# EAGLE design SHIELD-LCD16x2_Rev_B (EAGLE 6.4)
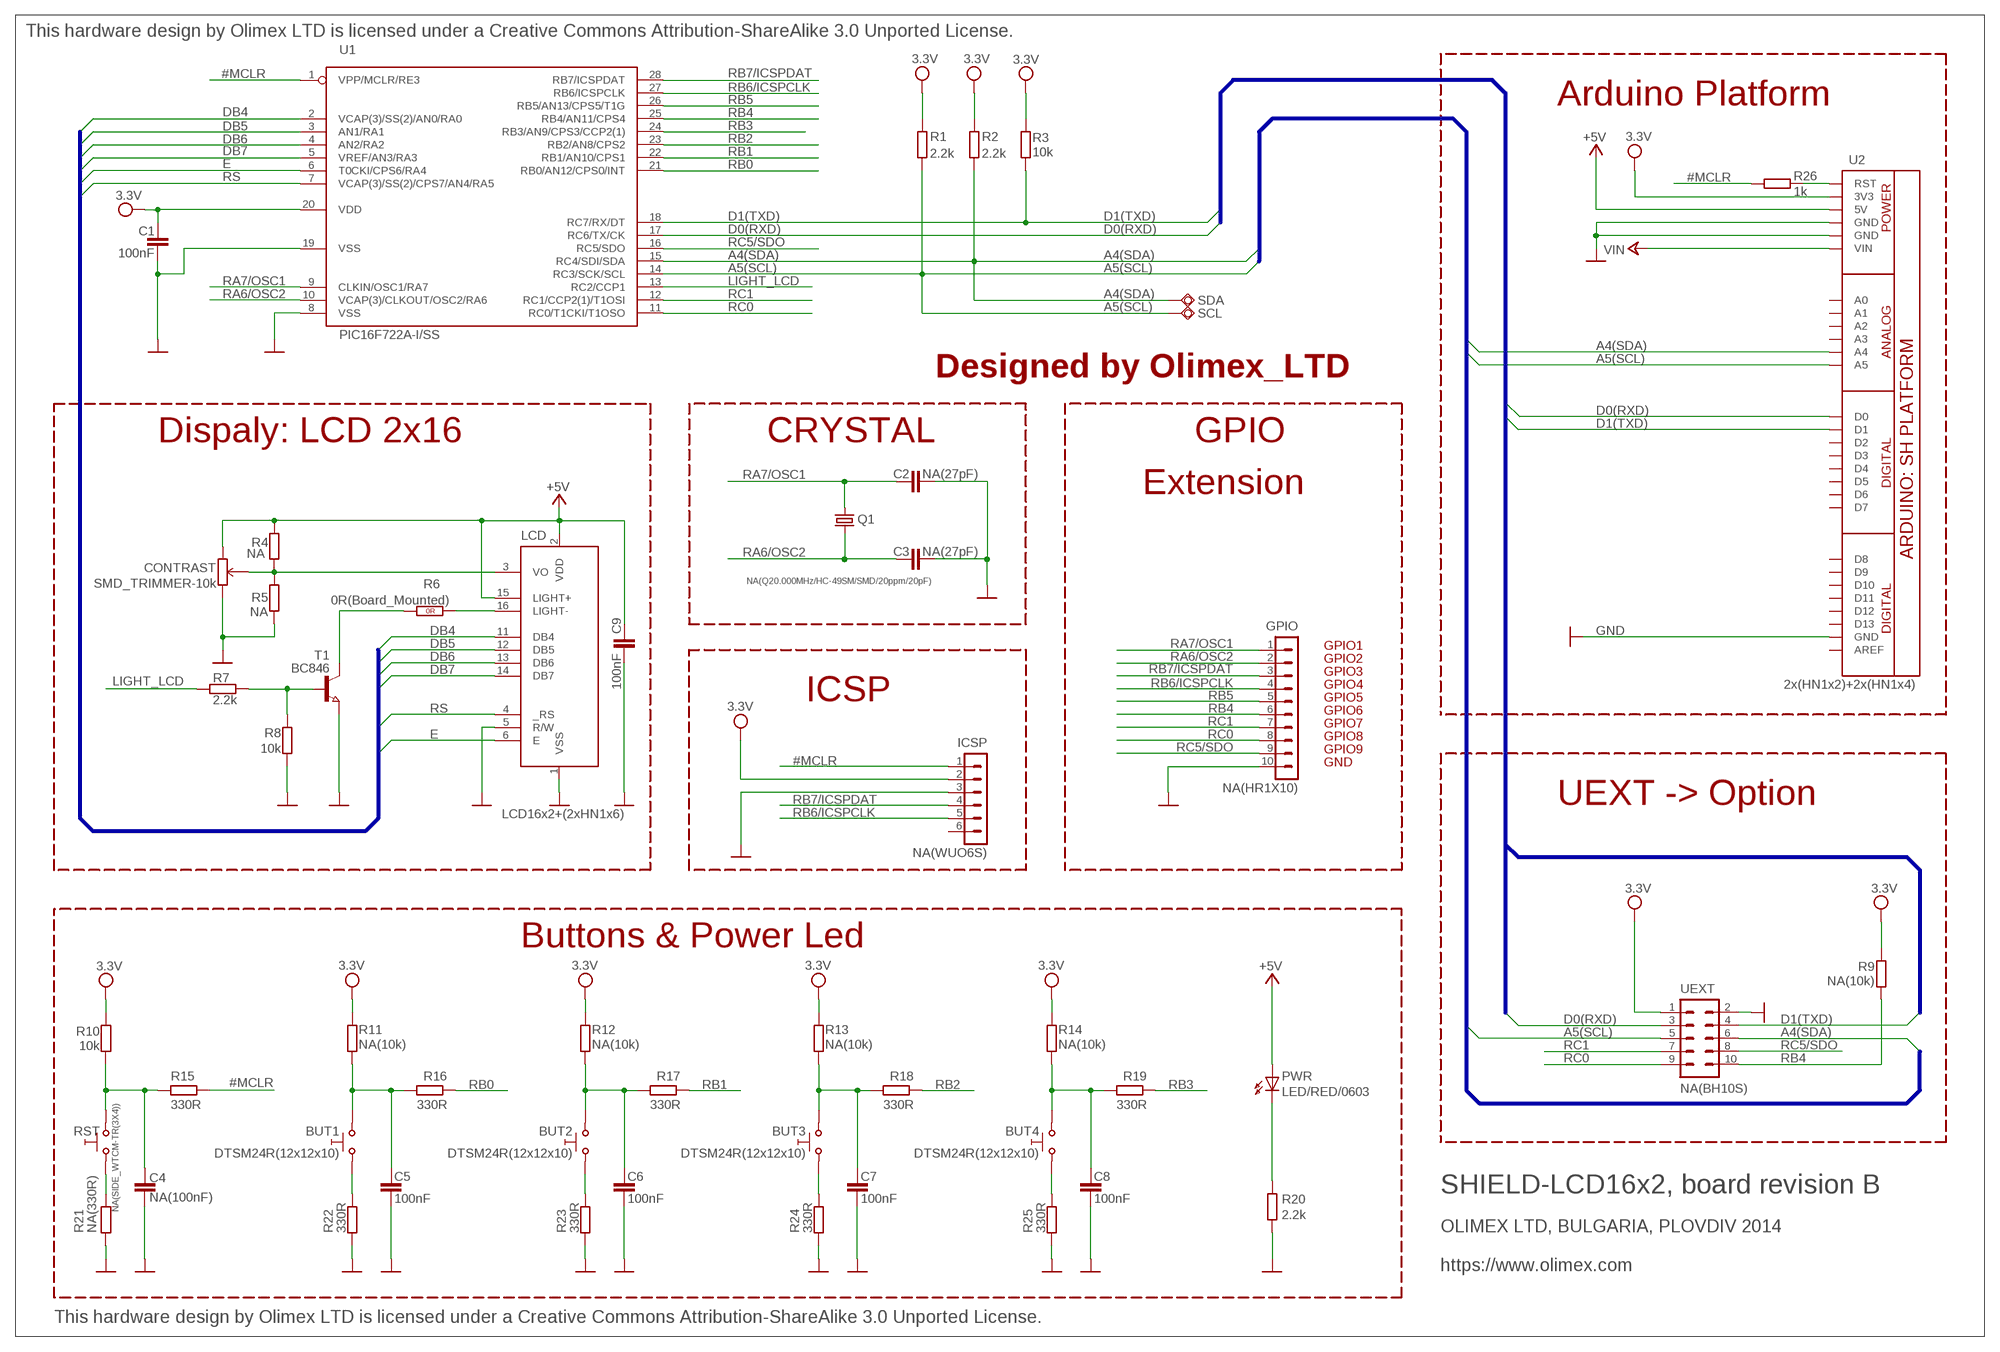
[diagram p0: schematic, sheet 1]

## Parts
BUT1  DTSM24R(12x12x10)  SW-TAKTSS  [SW_TAKT12X12SS]
BUT2  DTSM24R(12x12x10)  SW-TAKTSS  [SW_TAKT12X12SS]
BUT3  DTSM24R(12x12x10)  SW-TAKTSS  [SW_TAKT12X12SS]
BUT4  DTSM24R(12x12x10)  SW-TAKTSS  [SW_TAKT12X12SS]
C1  100nF  C-EUC0603_DWS  [C0603_DWS]
C2  NA(27pF)  C-EUC0603_DWS  [C0603_DWS]
C3  NA(27pF)  C-EUC0603_DWS  [C0603_DWS]
C4  NA(100nF)  C-EUC0603_DWS  [C0603_DWS]
C5  100nF  C-EUC0603_DWS  [C0603_DWS]
C6  100nF  C-EUC0603_DWS  [C0603_DWS]
C7  100nF  C-EUC0603_DWS  [C0603_DWS]
C8  100nF  C-EUC0603_DWS  [C0603_DWS]
C9  100nF  C-EUC0603_DWS  [C0603_DWS]
CONTRAST  SMD_TRIMMER-10k  TRSMD  [RTRIM3202]
GPIO  NA(HR1X10)  CON10HN1X10  [HN1X10]
ICSP  NA(WUO6S)  CON6WUO6S  [WU06S]
LCD  LCD16x2+(2xHN1x6)  LCD_MIN_LIGHT  [LCD_MIN_LIGHT]
PWR  LED/RED/0603  LED0603DWS  [LED-0603]
Q1  NA(Q20.000MHz/HC-49SM/SMD/20ppm/20pF)  HC49/S1  [HC49/SMD2_THIN]
R1  2.2k  R-EU_R0603_5MIL_DWS  [R0603_5MIL_DWS]
R2  2.2k  R-EU_R0603_5MIL_DWS  [R0603_5MIL_DWS]
R3  10k  R-EU_R0603_5MIL_DWS  [R0603_5MIL_DWS]
R4  NA  R-EU_R0603_5MIL_DWS  [R0603_5MIL_DWS]
R5  NA  R-EU_R0603_5MIL_DWS  [R0603_5MIL_DWS]
R6  0R(Board_Mounted)  R_0R0R(NA)  [0603_0R]
R7  2.2k  R-EU_R0603_5MIL_DWS  [R0603_5MIL_DWS]
R8  10k  R-EU_R0603_5MIL_DWS  [R0603_5MIL_DWS]
R9  NA(10k)  R-EU_R0603_5MIL_DWS  [R0603_5MIL_DWS]
R10  10k  R-EU_R0603_5MIL_DWS  [R0603_5MIL_DWS]
R11  NA(10k)  R-EU_R0603_5MIL_DWS  [R0603_5MIL_DWS]
R12  NA(10k)  R-EU_R0603_5MIL_DWS  [R0603_5MIL_DWS]
R13  NA(10k)  R-EU_R0603_5MIL_DWS  [R0603_5MIL_DWS]
R14  NA(10k)  R-EU_R0603_5MIL_DWS  [R0603_5MIL_DWS]
R15  330R  R-EU_R0603_5MIL_DWS  [R0603_5MIL_DWS]
R16  330R  R-EU_R0603_5MIL_DWS  [R0603_5MIL_DWS]
R17  330R  R-EU_R0603_5MIL_DWS  [R0603_5MIL_DWS]
R18  330R  R-EU_R0603_5MIL_DWS  [R0603_5MIL_DWS]
R19  330R  R-EU_R0603_5MIL_DWS  [R0603_5MIL_DWS]
R20  2.2k  R-EU_R0603_5MIL_DWS  [R0603_5MIL_DWS]
R21  NA(330R)  R-EU_R0603_5MIL_DWS  [R0603_5MIL_DWS]
R22  330R  R-EU_R0603_5MIL_DWS  [R0603_5MIL_DWS]
R23  330R  R-EU_R0603_5MIL_DWS  [R0603_5MIL_DWS]
R24  330R  R-EU_R0603_5MIL_DWS  [R0603_5MIL_DWS]
R25  330R  R-EU_R0603_5MIL_DWS  [R0603_5MIL_DWS]
R26  1k  R-EU_R0603_5MIL_DWS  [R0603_5MIL_DWS]
RST  NA(SIDE_WTCM-TR(3X4))  SW-TAKTSIDE_WTCM-TR(3X4)  [SW_TAKT3X4]
SCL  TESTPAD40/70  [TESTPAD]
SDA  TESTPAD40/70  [TESTPAD]
T1  BC846  NPN-TRANSISTOR_SOT23  [SOT23]
U1  PIC16F722A-I/SS  [SSOP28]
U2  2x(HN1x2)+2x(HN1x4)  ARDUINO_SH_PLATFORMLCD-PLATFORM  [ARDUINO_SH_LCD-PLATFORM]
UEXT  NA(BH10S)  ML10SMD  [ML10_PADS]

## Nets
#MCLR: ICSP.1 R15.2 R26.1 U1.1(VPP/MCLR/RE3)
+5V: C9.2 CONTRAST.2 LCD.2(VDD) LCD.15(LIGHT+) PWR.A R4.2 U2.5V
+24V: U2.VIN ; supply symbol labelled VIN
A4(SDA): R2.2 SDA.P$1(PP) U1.15(RC4/SDI/SDA) U2.A4 UEXT.6
A5(SCL): R1.2 SCL.P$1(PP) U1.14(RC3/SCK/SCL) U2.A5 UEXT.5
D0(RXD): U1.17(RC6/TX/CK) U2.D0 UEXT.3
D1(TXD): R3.1 U1.18(RC7/RX/DT) U2.D1 UEXT.4
DB4: LCD.11(DB4) U1.2(VCAP(3)/SS(2)/AN0/RA0)
DB5: LCD.12(DB5) U1.3(AN1/RA1)
DB6: LCD.13(DB6) U1.4(AN2/RA2)
DB7: LCD.14(DB7) U1.5(VREF/AN3/RA3)
E: LCD.6(E) U1.6(T0CKI/CPS6/RA4)
GND [pwr]: C1.1 C2.2 C3.2 C4.2 C5.2 C6.2 C7.2 C8.2 C9.1 CONTRAST.1 GPIO.10 ICSP.3 LCD.1(VSS) LCD.5(R/W) R5.1 R8.1 R20.1 R21.1 R22.1 R23.1 R24.1 R25.1 T1.2(E) U1.8(VSS) U1.19(VSS) U2.GND U2.GND@1(GND) U2.GND@2(GND) UEXT.2
LIGHT-: LCD.16(LIGHT-) R6.2(1.2)
LIGHT_LCD: R7.2 U1.13(RC2/CCP1)
N$1: BUT2.P$1 R23.2
N$2: C4.1 R10.1 R15.1 RST.2_1
N$3: BUT2.P$2 C6.1 R12.2 R17.1
N$4: BUT1.P$2 C5.1 R11.2 R16.1
N$5: BUT3.P$1 R24.2
N$6: BUT3.P$2 C7.1 R13.2 R18.1
N$7: BUT4.P$1 R25.2
N$8: BUT4.P$2 C8.1 R14.2 R19.1
N$9: R26.2 U2.RST
N$11 [pwr]: R21.2 RST.1_1
N$12: BUT1.P$1 R22.2
N$100: PWR.C R20.2
N$112: R7.1 R8.2 T1.1(B)
N$114: R6.1(1.1) T1.3(C)
RA6/OSC2: C3.1 GPIO.2 Q1.2 U1.10(VCAP(3)/CLKOUT/OSC2/RA6)
RA7/OSC1: C2.1 GPIO.1 Q1.1 U1.9(CLKIN/OSC1/RA7)
RB0: R16.2 U1.21(RB0/AN12/CPS0/INT)
RB1: R17.2 U1.22(RB1/AN10/CPS1)
RB2: R18.2 U1.23(RB2/AN8/CPS2)
RB3: R19.2 U1.24(RB3/AN9/CPS3/CCP2(1))
RB4: GPIO.6 R9.1 U1.25(RB4/AN11/CPS4) UEXT.10
RB5: GPIO.5 U1.26(RB5/AN13/CPS5/T1G)
RB6/ICSPCLK: GPIO.4 ICSP.5 U1.27(RB6/ICSPCLK)
RB7/ICSPDAT: GPIO.3 ICSP.4 U1.28(RB7/ICSPDAT)
RC0: GPIO.8 U1.11(RC0/T1CKI/T1OSO) UEXT.9
RC1: GPIO.7 U1.12(RC1/CCP2(1)/T1OSI) UEXT.7
RC5/SDO: GPIO.9 U1.16(RC5/SDO) UEXT.8
RS: LCD.4(_RS) U1.7(VCAP(3)/SS(2)/CPS7/AN4/RA5)
VCC: C1.2 ICSP.2 R1.1 R2.1 R3.2 R9.2 R10.2 R11.1 R12.1 R13.1 R14.1 U1.20(VDD) U2.3V3 UEXT.1 ; supply symbol labelled 3.3V
VO: CONTRAST.3 LCD.3(VO) R4.1 R5.2
Unconnected: ICSP.6 U2.A0 U2.A1 U2.A2 U2.A3 U2.AREF U2.D2 U2.D3 U2.D4 U2.D5 U2.D6 U2.D7 U2.D8 U2.D9 U2.D10 U2.D11 U2.D12 U2.D13

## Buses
A[0..3],A4(SDA),A5(SCL)
D0(RXD),D1(TXD),D2(BUT),D[3..7]
P0.4/SCK0,P0.5/MISO0,P0.6/MOSI0,P0.7/SSEL0

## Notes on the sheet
- This hardware design by Olimex LTD is licensed under a Creative Commons Attribution-ShareAlike 3.0 Unported License.
- Arduino Platform
- Designed by Olimex_LTD
- Dispaly: LCD 2x16 | CRYSTAL | GPIO
- Extension
- GPIO1
- GPIO2
- GPIO3
- GPIO4
- ICSP | GPIO5
- GPIO6
- GPIO7
- GPIO8
- GPIO9
- GND
- UEXT -> Option
- Buttons & Power Led
- SHIELD-LCD16x2, board revision B
- OLIMEX LTD, BULGARIA, PLOVDIV 2014
- https://www.olimex.com
- This hardware design by Olimex LTD is licensed under a Creative Commons Attribution-ShareAlike 3.0 Unported License.

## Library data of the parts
BUT1-BUT4 RST = gogo:SW-TAKT
C1-C9 = rcl:C-EU: CAPACITOR, European symbol
CONTRAST = DOUBLE-SIDE:TR: TRIMMER
GPIO = Penko:CON10
ICSP = Penko:CON6: CONNECTORS - 6 PINS
LCD = D-SIDE:LCD_MIN_LIGHT
PWR = DOUBLE-SIDE:LED
Q1 = crystal:HC49/S: CRYSTAL
R1-R5 R7-R26 = rcl:R-EU_: RESISTOR, European symbol
R6 = OLIMEX_DISCRET:R_0R
SCL SDA = gogo:TESTPAD: drill 40mils, diameter 70mils
T1 = semicon-smd-ipc:NPN-TRANSISTOR_: NPN TRANSISTOR
U1 = OLIMEX_IC:PIC16F722A: PIC16F722A Description: 28-Pin Flash Microcontrollers with nanoWatt XLP Technology
U2 = OLIMEX_CASES:ARDUINO_SH_PLATFORM
UEXT = con-harting-ml:ML10: HARTING

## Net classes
1 pwr: width 0.24 mm, clearance 0.24 mm

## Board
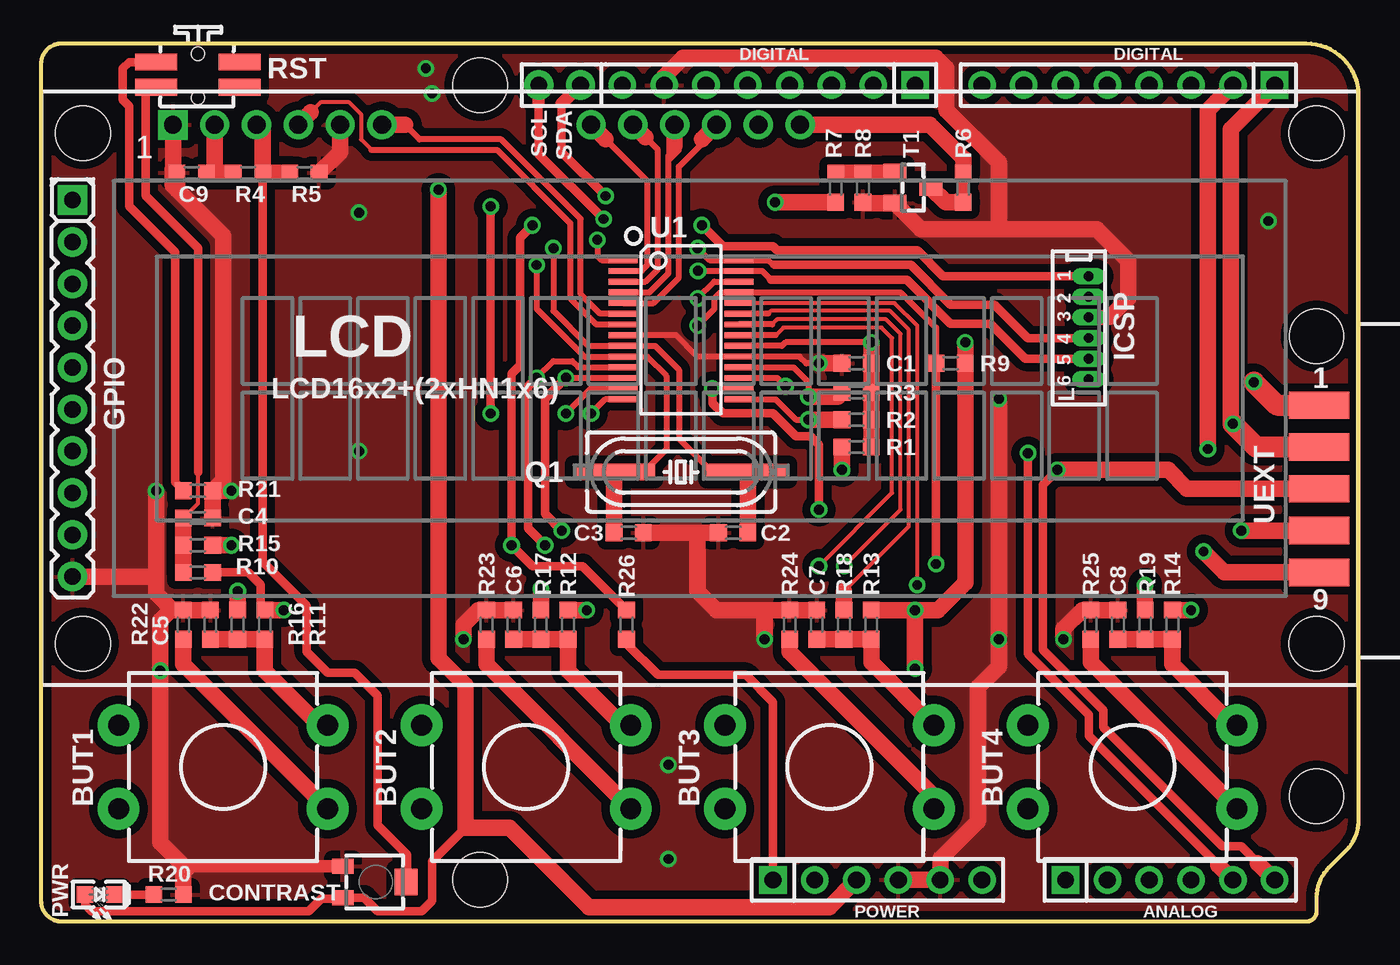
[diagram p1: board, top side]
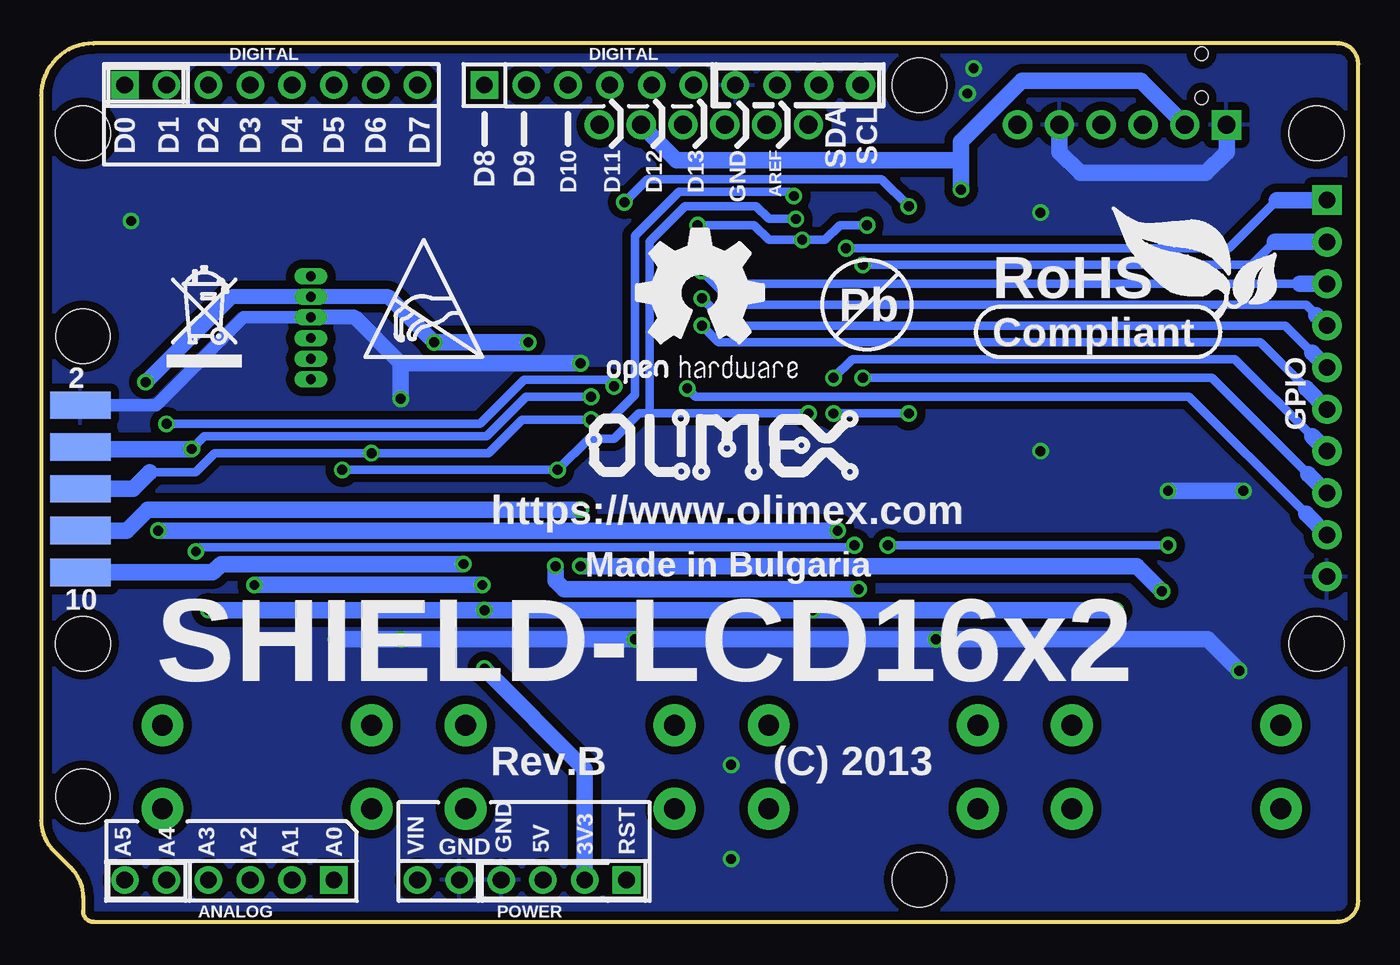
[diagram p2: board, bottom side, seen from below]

Size 80.01 x 53.34 mm. Coordinates in mm from the lower left corner, seen from the top.
Copper layers (1+16): Top 0.035mm / dielectric 1.5mm / Bottom 0.035mm
Design rules "default": minimum track width 10mil, minimum drill 0.6mm, track to track 8mil, track to pad 8mil, pad to pad 8mil, via to via 10mil, smd to smd 1mil, copper to edge 10mil, drill to drill 8mil, minimum pad ring 8mil, minimum via ring 8mil, stop-mask expansion 4mil, vias tented up to drill 25mil, thermal gap 20mil

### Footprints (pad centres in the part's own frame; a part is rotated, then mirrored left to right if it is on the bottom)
SW_TAKT12X12SS = drill 1.27 pad 2.54: P$1 -2.54,-6.35; P$2 2.54,-6.35; P$3 2.54,6.35; P$4 -2.54,6.35
C0603_DWS = smd 1.016 x 1.016: 1 -0.889,0; 2 0.889,0
RTRIM3202 = smd 0.9 x 1.3: 1 -0.95,-2.004; 2 0.95,-2.004 | smd 1.6 x 1.4: 3 0,1.854
HN1X10 = drill 1 pad 1.778 square: 1 -11.43,0 | drill 1 pad 1.778: 2 -8.89,0; 3 -6.35,0; 4 -3.81,0; 5 -1.27,0; 6 1.27,0; 7 3.81,0; 8 6.35,0; 9 8.89,0; 10 11.43,0
WU06S = drill 0.6 pad 0.991 long: 1 -3.125,0; 2 -1.875,0; 3 -0.625,0; 4 0.625,0; 5 1.875,0; 6 3.125,0
LCD_MIN_LIGHT = drill 1.092 pad 1.778 square: 1 -32,16 | drill 1.092 pad 1.778: 2 -29.464,16.002; 3 -26.924,16.002; 4 -24.384,16.002; 5 -21.844,16.002; 6 -19.304,16.002; 11 -6.604,16.002; 12 -4.064,16.002; 13 -1.524,16.002; 14 1.016,16.002; 15 3.556,16.002; 16 6.096,16.002 | hole 3.302: -37.465,15.494; 37.465,15.494; 37.465,-15.494; -37.465,-15.494
LED-0603 = smd 1.016 x 1.016: A 0.889,0; C -0.889,0
HC49/SMD2_THIN = smd 5 x 1: 1 -4.064,0; 2 4.064,0
R0603_5MIL_DWS = smd 1.016 x 1.016: 1 -0.889,0; 2 0.889,0
0603_0R = smd 1.016 x 1.016: 1 -0.889,0; 2 0.889,0
SW_TAKT3X4 = smd 2.54 x 1.016: 1_1 -2.54,0.762; 1_2 2.54,0.762; 2_1 -2.54,-0.762; 2_2 2.54,-0.762 | hole 0.8: 0,-1.397; 0,1.27
TESTPAD = drill 1.016 pad 1.778: P$1 0,0
SOT23 = smd 1 x 1.4: 1 -0.95,-1.1; 2 0.95,-1.1; 3 0,1.1
SSOP28 = smd 0.35 x 1.75: 1 -4.225,-3.525; 2 -3.575,-3.525; 3 -2.925,-3.525; 4 -2.275,-3.525; 5 -1.625,-3.525; 6 -0.975,-3.525; 7 -0.325,-3.525; 8 0.325,-3.525; 9 0.975,-3.525; 10 1.625,-3.525; 11 2.275,-3.525; 12 2.925,-3.525; 13 3.575,-3.525; 14 4.225,-3.525; 15 4.225,3.525; 16 3.575,3.525; 17 2.925,3.525; 18 2.275,3.525; 19 1.625,3.525; 20 0.975,3.525; 21 0.325,3.525; 22 -0.325,3.525; 23 -0.975,3.525; 24 -1.625,3.525; 25 -2.275,3.525; 26 -2.925,3.525; 27 -3.575,3.525; 28 -4.225,3.525
ARDUINO_SH_LCD-PLATFORM = drill 1.016 pad 1.676: 3V3 46.99,2.54; 5V 49.53,2.54; A1 64.77,2.54; A2 67.31,2.54; A3 69.85,2.54; A4 72.39,2.54; A5 74.93,2.54; AREF 35.306,50.8; D1 72.39,50.8; D2 69.85,50.8; D3 67.31,50.8; D4 64.77,50.8; D5 62.23,50.8; D6 59.69,50.8; D7 57.15,50.8; D9 50.546,50.8; D10 48.006,50.8; D11 45.466,50.8; D12 42.926,50.8; D13 40.386,50.8; GND 52.07,2.54; GND@1 54.61,2.54; GND@2 37.846,50.8; VIN 57.15,2.54 | drill 1.016 pad 1.676 square: A0 62.23,2.54; D0 74.93,50.8; D8 53.086,50.8; RST 44.45,2.54 | hole 3.3: 77.47,35.56; 77.47,7.62; 26.67,50.8; 26.67,2.54
ML10_PADS = smd 1.651 x 3.683: 1 -5.08,-0.229; 3 -2.54,-0.229; 5 0,-0.229; 7 2.54,-0.229; 9 5.08,-0.229 | smd 1.651 x 3.683 bottom: 2 -5.08,-0.229; 4 -2.54,-0.229; 6 0,-0.229; 8 2.54,-0.229; 10 5.08,-0.229

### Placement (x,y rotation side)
BUT1  11.05,9.4 90 top
BUT2  29.46,9.4 90 top
BUT3  47.88,9.4 90 top
BUT4  66.29,9.4 90 top
C1  49.53,33.91 0 top
C2  42.04,23.62 180 top
C3  35.69,23.62 0 top
C4  9.53,24.51 0 top
C5  10.29,18.03 90 top
C6  28.7,18.03 90 top
C7  47.12,18.03 90 top
C8  65.41,18.03 90 top
C9  9.14,45.47 0 top
CONTRAST  20.32,2.41 270 top
GPIO  1.91,32.38 270 top
ICSP  63.63,36.07 270 top
LCD  40.01,32.38 0 top
PWR  3.56,1.65 180 top
Q1  38.86,27.3 180 top
R1  49.53,28.83 180 top
R2  49.53,30.48 180 top
R3  49.53,32.13 0 top
R4  12.57,45.47 180 top
R5  16,45.47 180 top
R6  56.01,44.58 90 top
R7  48.26,44.58 270 top
R8  49.91,44.58 90 top
R9  55.24,33.91 0 top
R10  9.53,21.21 0 top
R11  13.59,18.03 270 top
R12  32,18.03 270 top
R13  50.42,18.03 270 top
R14  68.71,18.03 270 top
R15  9.53,22.86 0 top
R16  11.94,18.03 90 top
R17  30.35,18.03 90 top
R18  48.77,18.03 90 top
R19  67.06,18.03 90 top
R20  7.75,1.65 180 top
R21  9.53,26.16 180 top
R22  8.64,18.03 270 top
R23  27.05,18.03 270 top
R24  45.47,18.03 270 top
R25  63.75,18.03 270 top
R26  35.56,18.03 270 top
RST  9.53,51.44 0 top
SCL  30.23,50.8 180 top
SDA  32.77,50.8 180 top
T1  52.96,44.58 270 top
U1  38.86,35.94 270 top
U2  0,0 0 top
U$2  [ESD_SYMBOL]  60.33,34.29 0 bottom
U$3  [RECYCLE_BIN1/8]  72.39,33.66 0 bottom
U$4  [LOGO-OPENHARDWARE_8X8]  40.01,38.1 0 bottom
U$5  [OLIMEX1_V]  29.21,26.67 0 bottom
U$9  [PB]  29.84,37.47 0 bottom
U$14  [ROHS]  22.23,34.92 0 bottom
UEXT  77.85,26.29 270 top

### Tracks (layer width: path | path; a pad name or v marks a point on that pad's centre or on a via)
#MCLR  (via drill 0.6)
  Top 0.356: v33.78,41.4 33.78,40.42 34.04,40.17 U1.1
  Top 0.508: v29.84,42.29 29.08,41.53 29.08,33.78 28.57,33.27 v28.57,22.86 29.84,21.59 32.89,21.59 R26.1 | ICSP.1 54.79,39.19 53.21,40.77 44.7,40.77 44.45,41.02 41.4,41.02 v40.13,42.29
  Top 1.016: R15.2 v11.56,22.86
  Bottom 0.508: v29.84,42.29 31.5,42.29 32.38,41.4 v33.78,41.4 35.81,41.4 36.7,42.29 v40.13,42.29 | v11.56,22.86 v28.57,22.86
+5V  (via drill 0.6)
  Top 0.508: PWR.A 2.67,1.02 3.05,0.64 16.26,0.64 17.02,1.4 18.32,1.4 CONTRAST.2 19.62,1.46 20.45,0.64 23.11,0.64 23.75,1.27 23.75,3.68 25.78,5.71
  Top 1.016: LCD.2 10.54,45.47 | 10.54,45.47 C9.2 | 10.54,45.47 R4.2 | U2.5V 47.88,0.89 33.27,0.89 28.45,5.71 25.78,5.71 25.78,14.35 24.13,16 v24.13,44.45
  Bottom 1.016: LCD.2 13.21,51.05 20.45,51.05 24.13,47.37 24.13,46.23 | v24.13,44.45 24.13,46.23 | 24.13,46.23 41.4,46.23 LCD.15
A4(SDA)  (via drill 0.6)
  Top 0.356: U1.15 44.61,31.72 45.85,30.48 v46.61,30.48
  Top 0.508: 31.62,49.66 31.62,46.74 v34.29,44.07 | 71.5,3.43 63.63,11.3 63.63,12.57 59.94,16.26 v59.94,28.45
  Top 0.762: 31.62,49.66 SDA.P$1
  Top 1.016: v46.61,30.48 R2.2 | 71.5,3.43 U2.A4
  Bottom 0.508: v34.29,44.07 34.54,44.32 41.27,44.32 43.94,41.66 43.94,32 45.47,30.48 v46.61,30.48 50.8,30.48 52.83,28.45 v59.94,28.45 69.47,28.45 70.61,27.3 73.41,27.3
  Bottom 1.016: 73.41,27.3 74.42,26.29 UEXT.6
A5(SCL)  (via drill 0.6)
  Top 0.356: U1.14 34.26,31.72 v33.4,30.86
  Top 0.508: 30.23,49.66 30.23,46.61 v34.16,42.67 | 73.91,3.56 72.9,4.57 71.75,4.57 64.52,11.81 64.52,12.83 60.83,16.51 60.83,26.54 v61.72,27.43
  Top 0.762: 30.23,49.66 SCL.P$1
  Top 1.016: v48.64,27.43 R1.2 | 73.91,3.56 U2.A5 | v61.72,27.43 68.45,27.43 69.6,26.29 UEXT.5
  Bottom 0.508: v33.4,30.86 43.05,30.86 | 43.05,30.86 43.69,30.86 45.21,29.34 46.74,29.34 v48.64,27.43 v61.72,27.43 | v34.16,42.67 35.81,42.67 36.58,43.43 40.89,43.43 43.05,41.27 43.05,30.86
D0(RXD)  (via drill 0.6)
  Top 0.356: U1.17 44.71,33.02 v45.21,32.51
  Top 1.016: v72.39,30.23 72.26,30.35 72.26,48.13 U2.D0
  Top 1.27: v72.39,30.23 73.79,28.83 UEXT.3
  Bottom 0.508: v45.21,32.51 45.59,32.89 50.67,32.89 53.34,30.23 v72.39,30.23
D1(TXD)  (via drill 0.6)
  Top 0.356: U1.18 45.71,33.67 46.61,32.77 v46.61,31.88
  Top 1.016: v70.87,28.7 70.87,49.28 71.37,49.78 U2.D1 | v46.61,31.88 48.39,31.88 R3.1
  Bottom 0.508: v46.61,31.88 50.55,31.88 52.96,29.46 70.1,29.46 v70.87,28.7
  Bottom 1.016: v70.87,28.7 77.62,28.7 UEXT.4
DB4
  Top 0.356: 34.29,47.5 36.83,44.96 36.83,39.88 36.47,39.52 U1.2
  Top 1.016: 34.29,47.5 LCD.11
DB5
  Top 0.356: 36.7,47.62 37.47,46.86 37.47,39.62 36.71,38.87 U1.3
  Top 1.016: 36.7,47.62 LCD.12
DB6
  Top 0.254: 38.1,46.48 38.1,47.12 38.48,47.12
  Top 0.356: U1.4 36.95,38.22 38.1,39.37 38.1,46.23 | 38.1,46.23 38.1,46.48 38.48,46.86 | 38.1,46.23 38.73,46.86
  Top 1.016: 38.48,47.12 LCD.13
DB7
  Top 0.356: U1.5 37.19,37.57 38.73,39.12 38.73,45.85 40.13,47.24 40.13,47.5
  Top 1.016: 40.13,47.5 LCD.14
E
  Top 0.356: U1.6 33.95,36.92 32.77,38.1 32.77,42.67 27.94,47.5 22.99,47.5 22.1,48.39
  Top 1.016: 22.1,48.39 LCD.6
GND  (via drill 0.6)
  Top 0.254: 42.29,34.29 42.29,34.32 U1.19
  Top 0.356: U1.8 38.55,35.62 39.85,34.32 U1.19 46.08,34.32 46.48,33.91 C1.1
  Top 0.762: CONTRAST.1 9.21,3.36 8.64,2.79
  Top 0.914: ICSP.3 64.89,36.69 66.04,37.85
  Top 1.016: C7.2 R24.1 43.94,18.92 | C8.2 R25.1 63.25,18.92 62.1,17.78 v62.1,17.14 | R5.1 18.16,46.74 LCD.5 | U2.GND U2.GND@1 54.61,3.81 56.9,6.1 56.9,14.22 58.17,15.49 v58.17,17.14 v58.17,31.75 | C5.2 R22.1 8,18.92 | C6.2 R23.1 26.54,18.92 25.65,18.03 v25.65,17.14 | 39.88,23.62 C2.2 | R21.1 C4.2 | C9.1 8,45.72 8,44.7 8.26,44.45 | 8,18.92 7.87,18.92 7.24,18.29 v7.24,15.24 7.24,4.83 8.64,3.43 8.64,2.79 R20.1 | v43.94,17.14 43.94,18.92 | 8.26,44.45 C9.1 | 8.26,44.45 11.05,41.66 11.05,26.8 R21.1 | v11.56,26.16 R21.1 | 6.99,20.95 v6.99,26.16 | 6.99,20.95 GPIO.10 | 6.99,20.95 6.99,19.94 8,18.92 | U2.GND@2 37.85,51.31 38.99,52.45 54.36,52.45 54.99,51.82 54.99,49.28 58.17,46.1 58.17,42.04 58.29,42.04 | 58.29,42.04 64.14,42.04 66.04,40.13 66.04,37.85 | v47.24,33.91 C1.1 | 39.88,23.62 C3.2 | 43.94,18.92 41.02,18.92 39.88,20.07 39.88,23.62 | LCD.1 8.01,45.72 C9.1 | R8.1 49.97,43.63 T1.2 53.45,42.04 58.29,42.04
  Bottom 0.762: UEXT.2 73.03,31.37 67.7,36.69 ICSP.3
  Bottom 0.914: ICSP.3 60.95,36.69 58.17,33.91
  Bottom 1.016: LCD.5 18.16,46.74 R5.1 9.27,45.47 8,46.74 LCD.1 | v7.24,15.24 9.14,17.14 v25.65,17.14 v43.94,17.14 v58.17,17.14 v62.1,17.14 | v6.99,26.16 v11.56,26.16 | v47.24,33.91 58.17,33.91 v58.17,31.75 | LCD.1 | LCD.1
  other vias: 74.55,42.55 19.3,43.05 19.3,28.57 38.1,9.53 38.1,3.81 23.37,51.82 23.75,50.29
  pour Top (isolate 0.508, rank 4): -2.54,55.88 -2.54,-2.54 83.82,-2.54 83.82,55.88
  pour Bottom (isolate 0.508, rank 4): -5.08,58.42 -5.08,-5.08 86.36,-5.08 86.36,58.42
LIGHT-
  Top 1.016: R6.2 56.01,46.35 53.98,48.39 LCD.16
LIGHT_LCD  (via drill 0.6)
  Top 0.356: U1.13 33.38,32.37 v31.88,30.86
  Top 0.508: v27.3,30.86 v27.3,43.43
  Top 1.016: v44.58,43.69 R7.2
  Bottom 0.508: v44.58,43.69 43.18,45.09 28.96,45.09 v27.3,43.43 | v27.3,30.86 v31.88,30.86
N$1
  Top 1.016: R23.2 27.05,15.62 BUT2.P$1
N$2
  Top 0.254: C4.1 9.53,25.4 9.53,27.3
  Top 0.508: RST.2_1 6.35,50.67 6.35,44.07 9.53,40.89 9.53,27.3
  Top 1.016: C4.1 R15.1 R10.1
N$3
  Top 1.016: BUT2.P$2 35.31,11.94 32,15.24 R12.2 R17.1 C6.1
N$4
  Top 1.016: BUT1.P$2 16.89,11.94 13.59,15.24 R11.2 R16.1 C5.1
N$5
  Top 1.016: R24.2 45.47,16.38 54.23,7.62 BUT3.P$1
N$6
  Top 1.016: BUT3.P$2 50.42,15.75 R13.2 R18.1 C7.1
N$7
  Top 1.016: BUT4.P$1 63.75,15.75 R25.2
N$8
  Top 1.016: BUT4.P$2 72.39,11.94 68.71,15.62 R14.2 R19.1 C8.1
N$9
  Top 0.508: U2.RST 44.45,13.34 42.8,14.99 37.47,14.99 35.56,16.89 R26.2
N$11
  Top 0.508: RST.1_1 5.33,52.2 4.95,51.82 4.95,49.91 5.33,49.53 5.33,43.43 8.13,40.64 8.13,26.67 R21.2
N$12
  Top 1.016: R22.2 8.64,15.62 BUT1.P$1
N$100
  Top 0.508: PWR.C R20.2
N$112
  Top 0.254: 51.86,45.47 T1.1
  Top 1.016: R7.1 R8.2 51.86,45.47
N$114
  Top 1.016: T1.3 54.95,43.69 R6.1
RA6/OSC2  (via drill 0.6)
  Top 0.254: 35.31,34.29 35.31,34.32 U1.10
  Top 0.356: v30.1,39.88 30.1,37.21 32.99,34.32 35.31,34.32 | Q1.2 36.58,27.3 37.97,28.7 37.97,33.15 36.8,34.32 U1.10
  Top 1.016: Q1.2 C3.1
  Bottom 0.508: 5.08,41.27 6.48,39.88 v30.1,39.88
  Bottom 1.016: GPIO.2 5.08,41.27
RA7/OSC1  (via drill 0.6)
  Top 0.356: v31.11,40.89 31.11,37.08 33.23,34.97 U1.9 37.3,34.97 38.73,33.53 38.73,29.34 40.77,27.3 Q1.1
  Top 1.016: Q1.1 C2.1
  Bottom 0.508: v31.11,40.89 7.87,40.89 4.95,43.81
  Bottom 1.016: GPIO.1 4.95,43.81
RB0  (via drill 0.6)
  Top 0.254: v47.24,21.59 51.69,26.04 51.69,35.43 51.05,36.07 45.09,36.07 44.63,35.62
  Top 0.356: 44.63,35.62 U1.21
  Top 1.016: R16.2 v11.94,20.07
  Bottom 1.016: v11.94,20.07 13.46,21.59 v47.24,21.59
RB1  (via drill 0.6)
  Top 0.254: v48.77,21.59 52.2,25.02 52.2,35.69 51.31,36.58 44.7,36.58 44.39,36.27
  Top 0.356: 44.39,36.27 U1.22
  Top 1.016: R17.2 v30.35,20.19
  Bottom 1.016: v30.35,20.19 48.26,20.19 48.77,20.7 v48.77,21.59
RB2
  Top 0.254: 48.77,20.07 52.7,24 52.7,35.94 51.56,37.08 44.32,37.08 44.16,36.92
  Top 0.356: 44.16,36.92 U1.23
  Top 1.016: R18.2 48.77,20.07
RB3  (via drill 0.6)
  Top 0.254: v53.21,20.45 53.21,36.2 51.84,37.57 U1.24
  Top 1.016: v67.06,20.45 R19.2
  Bottom 1.016: v53.21,20.45 v67.06,20.45
RB4  (via drill 0.6)
  Top 0.356: v39.88,36.2 40.89,37.21 40.89,37.85 41.26,38.22 U1.25 52.21,38.22 54.36,36.07 R9.1
  Top 0.508: R9.1 v54.36,21.72
  Bottom 0.508: 3.17,32.38 5.97,35.18 38.86,35.18 v39.88,36.2
  Bottom 1.016: GPIO.6 3.17,32.38 | v54.36,21.72 69.09,21.72 69.6,21.21 UEXT.10
RB5  (via drill 0.6)
  Top 0.356: U1.26 40.9,38.87 v39.88,37.85
  Bottom 0.508: 2.79,34.54 4.45,36.2 38.23,36.2 v39.88,37.85
  Bottom 1.016: GPIO.5 2.79,34.54
RB6/ICSPCLK  (via drill 0.6)
  Top 0.254: U1.27 42.16,39.52
  Top 0.356: v39.9,39.52 U1.27 43.8,39.52 44.32,38.99
  Top 0.508: ICSP.5 59.79,34.19 57.66,36.32 55.24,36.32 52.58,38.99 44.32,38.99
  Bottom 0.508: 2.54,36.83 3.17,37.47 37.85,37.47 v39.9,39.52
  Bottom 1.016: GPIO.4 2.54,36.83
RB7/ICSPDAT  (via drill 0.6)
  Top 0.356: v39.88,40.89 40.61,40.17 U1.28 44.16,40.17 44.45,39.88 44.55,39.88
  Top 0.508: 44.55,39.88 52.83,39.88 55.24,37.47 57.91,37.47 59.93,35.44 ICSP.4
  Bottom 0.508: v39.88,40.89 39.75,40.89 37.59,38.73 3.56,38.73
  Bottom 1.016: GPIO.3 3.56,38.73
RC0  (via drill 0.6)
  Top 0.356: v30.1,33.02 31.11,34.04 32.26,34.04 32.63,33.67 U1.11
  Top 0.508: v30.1,33.02 29.59,32.51 29.59,23.88 v30.61,22.86
  Top 1.016: v70.61,22.48 71.88,21.21 UEXT.9
  Bottom 0.508: 3.05,27.18 8.89,33.02 v30.1,33.02 | v30.61,22.86 30.73,22.73 70.36,22.73 v70.61,22.48
  Bottom 1.016: GPIO.8 3.05,27.18
RC1  (via drill 0.6)
  Top 0.254: 35.31,33.02 U1.12
  Top 0.356: v31.88,33.02 35.31,33.02
  Top 0.508: v31.62,23.75 30.61,24.77 30.61,31.75 v31.88,33.02
  Top 1.016: v72.9,23.75 UEXT.7
  Bottom 0.508: 2.79,29.46 7.49,34.16 30.73,34.16 v31.88,33.02
  Bottom 1.016: GPIO.7 2.79,29.46 | v31.62,23.75 v72.9,23.75
RC5/SDO  (via drill 0.6)
  Top 0.254: 40.75,32.37 v40.77,32.38 40.79,32.37
  Top 0.356: 40.79,32.37 U1.16
  Top 0.508: v47.24,25.02 47.24,28.96 46.74,29.46 45.85,29.46 44.45,30.86 41.4,30.86 40.77,31.5 v40.77,32.38
  Bottom 0.508: 3.17,24.77 10.29,31.88 40.26,31.88 v40.77,32.38
  Bottom 1.016: GPIO.9 3.17,24.77 | v47.24,25.02 73.53,25.02 74.8,23.75 UEXT.8
RS
  Top 0.254: 20.07,46.86 19.43,47.5 19.43,49.02 18.67,49.78 17.02,49.78 16.38,49.15
  Top 0.356: U1.7 33.71,36.27 32.13,37.85 32.13,42.42 27.69,46.86 20.07,46.86
  Top 1.016: LCD.4 16.38,49.15
VCC  (via drill 0.6)
  Top 0.356: v50.42,35.18 45.21,35.18 45,34.97 U1.20
  Top 0.508: R10.2 12.57,21.21 13.34,20.45 13.34,19.05 13.72,19.05 R11.1
  Top 1.016: v50.42,35.18 C1.2 R3.2 R2.1 R1.1 | v53.09,18.92 R13.1 | v69.85,18.92 R14.1 | R11.1 v14.73,18.92 | v33.15,18.92 R12.1 | v53.09,18.92 v53.09,15.37 | v56.13,35.18 R9.2 56.13,20.57 54.48,18.92 v53.09,18.92
  Top 1.27: UEXT.1 75.06,31.37 v73.66,32.77
  Bottom 0.914: v56.13,35.18 58.9,37.94 ICSP.2 68.48,37.94 v73.66,32.77
  Bottom 1.016: U2.3V3 46.99,9.27 v53.09,15.37 | v69.85,18.92 v53.09,18.92 v33.15,18.92 v14.73,18.92 | v56.13,35.18 v50.42,35.18
VO
  Top 0.508: CONTRAST.3 22.23,2.41 22.23,4.06 20.45,5.84 20.45,13.72 19.05,15.11 17.4,15.11 16.13,16.38 16.13,19.18 13.46,21.84 R4.1
  Top 1.016: R5.2 R4.1 13.46,48.01 LCD.3

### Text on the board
Top: Da se fiksne v Gerbtool liniqata v top silk, koqto zastypva RST butona i konektorite
bNames: DIGITAL | DIGITAL | D7 | D6 | D5 | D4 | D3 | D2 | D1 | D0 | AREF | GND | D13 | D12 | D11 | D10 | D9 | D8 | https://www.olimex.com | Made in Bulgaria | SHIELD-LCD16x2 | (C) 2013 | Rev.B | RST | 3V3 | 5V | GND | GND | VIN | A0 | A1 | A2 | A3 | A4 | A5 | POWER | ANALOG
